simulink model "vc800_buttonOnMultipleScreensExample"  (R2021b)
settings: Solver=FixedStepDiscrete  StartTime=0.0  StopTime=10.0  FixedStep=0.01  RelTol=1e-3  EnableMultiTasking=on
PreLoadFcn:
  | try, model_open; catch, disp('Error occurred while executing model pre-load callback: model_open.m'); disp('Please assure that the MATLAB working directory is set to the model directory before opening.'); end
InitFcn:
  | try, model_open; catch, end
model workspace (MAT data in the model file):
  IOScreen_Label_XCoord = 1
  IOScreen_Row1_YCoord = 1
  IOScreen_Row2_YCoord = 12
  IOScreen_Value_XCoord = 110
  MainScreen_Row1_YCoord = 7
  MainScreen_Row2_YCoord = 23
  MainScreen_Symbols_XCoord = 1
  MainScreen_Units_XCoord = 69
  MainScreen_Value_XCoord = 64
undefined symbols (not defined in the file or in its folder): case, curr_screen, default, DISP, filtering, gesture, hex2dec, Mode, No, raptor_get_buildNum, raptor_get_safe_string, raptor_hwexp, raptor_xcp_function, Screens, VC800, Voltage
libraries: Raptor_display_lib x190, Raptor_lib x97, simulink_extras x11, Raptor_Datalogging_lib x10, simulink x2
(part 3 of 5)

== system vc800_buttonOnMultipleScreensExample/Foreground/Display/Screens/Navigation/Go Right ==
  Current Screen : Inport
  Action Port : ActionPort  ActionPortLabel=if(u1 == 3)
  About : Subsystem  TreatAsAtomicUnit=on
  DataLog : Subsystem  TreatAsAtomicUnit=on
  Default : Subsystem  TreatAsAtomicUnit=on
  Input : Subsystem  TreatAsAtomicUnit=on
  Main : Subsystem  TreatAsAtomicUnit=on
  Ouptut : Subsystem  TreatAsAtomicUnit=on
  Switch Case : SwitchCase  CaseConditions={1,2,3,4,5}
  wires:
  Current Screen/1 -> Switch Case/1
  Switch Case/1 -> Main/Action
  Switch Case/4 -> DataLog/Action
  Switch Case/5 -> About/Action
  Switch Case/2 -> Input/Action
  Switch Case/6 -> Default/Action
  Switch Case/3 -> Ouptut/Action

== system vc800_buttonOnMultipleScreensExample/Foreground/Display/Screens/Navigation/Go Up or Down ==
  note: Do Nothing when a "UP" or "DOWN" is performed
  Current Screen : Inport
  Action Port : ActionPort  ActionPortLabel=else
  Terminator : Terminator
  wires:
  Current Screen/1 -> Terminator/1

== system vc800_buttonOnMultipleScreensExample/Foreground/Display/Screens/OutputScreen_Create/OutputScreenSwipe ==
  note: This function is called when a swipe action occurs. The gesture input will provide the gesture detected: 0 = UP 1 = DOWN 2 = LEFT 3 = RIGHT
  OutputScreenSwipe : TriggerPort  TriggerType=function-call  IsSimulinkFunction=on  FunctionName=OutputScreenSwipe  FunctionVisibility=scoped  VariantControl=Variant  PortDimensions=1
  Constant : Constant  Value=3  OutDataTypeStr=uint8
  Function Caller : FunctionCaller  FunctionPrototype=Screens.Navigation(gesture,curr_screen)  InputArgumentSpecifications=<Enter example>  OutputArgumentSpecifications=<Enter example>
  gesture : ArgIn  OutDataTypeStr=uint8  ArgumentName=gesture
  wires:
  gesture/1 -> Function Caller/1
  Constant/1 -> Function Caller/2

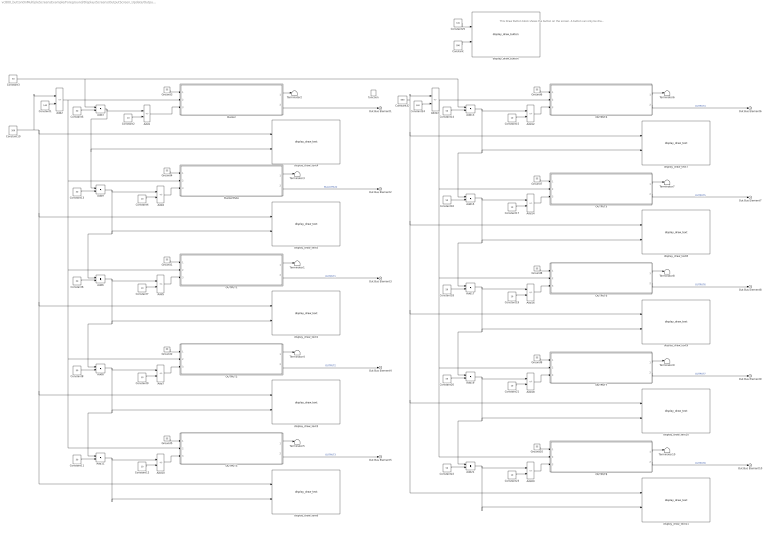
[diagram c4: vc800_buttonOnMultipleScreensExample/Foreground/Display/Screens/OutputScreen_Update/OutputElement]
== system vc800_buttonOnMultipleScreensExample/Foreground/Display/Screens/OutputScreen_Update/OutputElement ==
  note: This Draw Button block shows the button on the screen. A button can only be drawn once per screen.
  function : TriggerPort  TriggerType=function-call  VariantControl=Variant
  Add{1..2,4..5,7,10,12,14,16,18,20,22} (12 alike) : Sum  Inputs=+-
  Add{3,6,8..9,11,13,15,17,19,21} (10 alike) : Sum
  Buzzer : Subsystem  mask(Display Toggle){InitialCondition=0}
      mask prompts: InitialCondition "Initial Condition"
      mask help: Draws a toggle switch onto the screen that will hold either an off or an on state
  BuzzerMute : Subsystem  mask(Display Toggle){InitialCondition=0}
      mask prompts: InitialCondition "Initial Condition"
      mask help: Draws a toggle switch onto the screen that will hold either an off or an on state
  Constant : Constant  Value=390  OutDataTypeStr=Inherit: Inherit via back propagation
  Constant1 : Constant  Value=140  OutDataTypeStr=int32
  Constant10 : Constant  Value=200  OutDataTypeStr=int32
  Constant{3,5..6,8,11,13..14,16,18,20,22} (11 alike) : Constant  Value=50  OutDataTypeStr=int32
  Constant{2,4,7,9,12,15,17,19,21,23} (10 alike) : Constant  Value=10  OutDataTypeStr=int32
  Constant24 : Constant  Value=140  OutDataTypeStr=int32
  Constant25 : Constant  Value=720  OutDataTypeStr=Inherit: Inherit via back propagation
  Constant32 : Constant  Value=600  OutDataTypeStr=int32
  Ground{1..10} (10 alike) : Ground
  OUTPUT1 : Subsystem  mask(Display Toggle){InitialCondition=0}
      mask prompts: InitialCondition "Initial Condition"
      mask help: Draws a toggle switch onto the screen that will hold either an off or an on state
  OUTPUT2 : Subsystem  mask(Display Toggle){InitialCondition=0}
      mask prompts: InitialCondition "Initial Condition"
      mask help: Draws a toggle switch onto the screen that will hold either an off or an on state
  OUTPUT3 : Subsystem  mask(Display Toggle){InitialCondition=0}
      mask prompts: InitialCondition "Initial Condition"
      mask help: Draws a toggle switch onto the screen that will hold either an off or an on state
  OUTPUT4 : Subsystem  mask(Display Toggle){InitialCondition=0}
      mask prompts: InitialCondition "Initial Condition"
      mask help: Draws a toggle switch onto the screen that will hold either an off or an on state
  OUTPUT5 : Subsystem  mask(Display Toggle){InitialCondition=0}
      mask prompts: InitialCondition "Initial Condition"
      mask help: Draws a toggle switch onto the screen that will hold either an off or an on state
  OUTPUT6 : Subsystem  mask(Display Toggle){InitialCondition=0}
      mask prompts: InitialCondition "Initial Condition"
      mask help: Draws a toggle switch onto the screen that will hold either an off or an on state
  OUTPUT7 : Subsystem  mask(Display Toggle){InitialCondition=0}
      mask prompts: InitialCondition "Initial Condition"
      mask help: Draws a toggle switch onto the screen that will hold either an off or an on state
  OUTPUT8 : Subsystem  mask(Display Toggle){InitialCondition=0}
      mask prompts: InitialCondition "Initial Condition"
      mask help: Draws a toggle switch onto the screen that will hold either an off or an on state
  Terminator{1..10} (10 alike) : Terminator
  display_draw_button : Raptor_display_lib/Drawing Functions/display_draw_button  ButtonName='GoToAbout'
  display_draw_text1 : Raptor_display_lib/Drawing Functions/display_draw_text  textPort=off  textVal='OUTPUT1'  colorPort=off  col=FFFF  opacity=100  font=Future  fontFile=''  heightPort=off  height=20  hAlign=Left  vAlign=Top  spacing=0  layer=Background  pnPort=off
  display_draw_text10 : Raptor_display_lib/Drawing Functions/display_draw_text  textPort=off  textVal='OUTPUT7'  colorPort=off  col=FFFF  opacity=100  font=Future  fontFile=''  heightPort=off  height=20  hAlign=Left  vAlign=Top  spacing=0  layer=Background  pnPort=off
  display_draw_text11 : Raptor_display_lib/Drawing Functions/display_draw_text  textPort=off  textVal='OUTPUT8'  colorPort=off  col=FFFF  opacity=100  font=Future  fontFile=''  heightPort=off  height=20  hAlign=Left  vAlign=Top  spacing=0  layer=Background  pnPort=off
  display_draw_text3 : Raptor_display_lib/Drawing Functions/display_draw_text  textPort=off  textVal='OUTPUT2'  colorPort=off  col=FFFF  opacity=100  font=Future  fontFile=''  heightPort=off  height=20  hAlign=Left  vAlign=Top  spacing=0  layer=Background  pnPort=off
  display_draw_text4 : Raptor_display_lib/Drawing Functions/display_draw_text  textPort=off  textVal='Buzzer'  colorPort=off  col=FFFF  opacity=100  font=Future  fontFile=''  heightPort=off  height=20  hAlign=Left  vAlign=Top  spacing=0  layer=Background  pnPort=off
  display_draw_text5 : Raptor_display_lib/Drawing Functions/display_draw_text  textPort=off  textVal='Buzzer Mute'  colorPort=off  col=FFFF  opacity=100  font=Future  fontFile=''  heightPort=off  height=20  hAlign=Left  vAlign=Top  spacing=0  layer=Background  pnPort=off
  display_draw_text6 : Raptor_display_lib/Drawing Functions/display_draw_text  textPort=off  textVal='OUTPUT3'  colorPort=off  col=FFFF  opacity=100  font=Future  fontFile=''  heightPort=off  height=20  hAlign=Left  vAlign=Top  spacing=0  layer=Background  pnPort=off
  display_draw_text7 : Raptor_display_lib/Drawing Functions/display_draw_text  textPort=off  textVal='OUTPUT4'  colorPort=off  col=FFFF  opacity=100  font=Future  fontFile=''  heightPort=off  height=20  hAlign=Left  vAlign=Top  spacing=0  layer=Background  pnPort=off
  display_draw_text8 : Raptor_display_lib/Drawing Functions/display_draw_text  textPort=off  textVal='OUTPUT5'  colorPort=off  col=FFFF  opacity=100  font=Future  fontFile=''  heightPort=off  height=20  hAlign=Left  vAlign=Top  spacing=0  layer=Background  pnPort=off
  display_draw_text9 : Raptor_display_lib/Drawing Functions/display_draw_text  textPort=off  textVal='OUTPUT6'  colorPort=off  col=FFFF  opacity=100  font=Future  fontFile=''  heightPort=off  height=20  hAlign=Left  vAlign=Top  spacing=0  layer=Background  pnPort=off
  Out Bus Element{1..10} (10 alike) : Outport  VectorParamsAs1DForOutWhenUnconnected=off
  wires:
  Add20/1 -> OUTPUT8/3(y)
  Constant23/1 -> Add20/2
  Add19/1 -> Add18/1, Add21/1, display_draw_text10/2
  Add2/1 -> BuzzerMute/2(x), OUTPUT1/2(x), OUTPUT2/2(x), OUTPUT3/2(x), Buzzer/2(x)
  Constant10/1 -> Add2/1, display_draw_text5/1, display_draw_text1/1, display_draw_text3/1, display_draw_text6/1, display_draw_text4/1
  OUTPUT8/2(out) -> Out Bus Element10/1  "OUTPUT8"
  OUTPUT8/1(next) -> Terminator10/1
  Add21/1 -> display_draw_text11/2, Add20/1
  Ground10/1 -> OUTPUT8/1(prev)
  Constant22/1 -> Add21/2
  Constant20/1 -> Add19/2
  Ground9/1 -> OUTPUT7/1(prev)
  OUTPUT7/1(next) -> Terminator9/1
  OUTPUT7/2(out) -> Out Bus Element9/1  "OUTPUT7"
  Add17/1 -> display_draw_text9/2, Add19/1, Add16/1
  Constant21/1 -> Add18/2
  Add18/1 -> OUTPUT7/3(y)
  Add16/1 -> OUTPUT6/3(y)
  Constant19/1 -> Add16/2
  Add15/1 -> Add14/1, Add17/1, display_draw_text8/2
  OUTPUT6/2(out) -> Out Bus Element8/1  "OUTPUT6"
  OUTPUT6/1(next) -> Terminator8/1
  Ground8/1 -> OUTPUT6/1(prev)
  Constant18/1 -> Add17/2
  Constant16/1 -> Add15/2
  Ground7/1 -> OUTPUT5/1(prev)
  OUTPUT5/1(next) -> Terminator7/1
  OUTPUT5/2(out) -> Out Bus Element7/1  "OUTPUT5"
  Add13/1 -> Add15/1, display_draw_text7/2, Add12/1
  Constant17/1 -> Add14/2
  Add14/1 -> OUTPUT5/3(y)
  Add12/1 -> OUTPUT4/3(y)
  Constant15/1 -> Add12/2
  Add11/1 -> display_draw_text6/2, Add10/1
  OUTPUT4/2(out) -> Out Bus Element6/1  "OUTPUT4"
  OUTPUT4/1(next) -> Terminator6/1
  Ground6/1 -> OUTPUT4/1(prev)
  Constant14/1 -> Add13/2
  Constant11/1 -> Add11/2
  Ground5/1 -> OUTPUT3/1(prev)
  OUTPUT3/1(next) -> Terminator5/1
  OUTPUT3/2(out) -> Out Bus Element5/1  "OUTPUT3"
  Add8/1 -> display_draw_text3/2, Add11/1, Add7/1
  Constant12/1 -> Add10/2
  Add10/1 -> OUTPUT3/3(y)
  Add7/1 -> OUTPUT2/3(y)
  Constant9/1 -> Add7/2
  Add6/1 -> Add5/1, display_draw_text1/2, Add8/1
  OUTPUT2/2(out) -> Out Bus Element4/1  "OUTPUT2"
  OUTPUT2/1(next) -> Terminator4/1
  Ground2/1 -> OUTPUT2/1(prev)
  Constant8/1 -> Add8/2
  Constant6/1 -> Add6/2
  Ground1/1 -> OUTPUT1/1(prev)
  OUTPUT1/1(next) -> Terminator1/1
  OUTPUT1/2(out) -> Out Bus Element3/1  "OUTPUT1"
  Add9/1 -> Add6/1, display_draw_text5/2, Add4/1
  Constant7/1 -> Add5/2
  Add5/1 -> OUTPUT1/3(y)
  Add4/1 -> BuzzerMute/3(y)
  Constant4/1 -> Add4/2
  Add1/1 -> Buzzer/3(y)
  Constant2/1 -> Add1/2
  Constant5/1 -> Add3/2
  Add3/1 -> Add9/1, display_draw_text4/2, Add1/1
  Constant1/1 -> Add2/2
  Constant3/1 -> Add3/1, Add13/1
  Ground3/1 -> Buzzer/1(prev)
  Buzzer/1(next) -> Terminator2/1
  Buzzer/2(out) -> Out Bus Element1/1
  BuzzerMute/2(out) -> Out Bus Element2/1  "BuzzerMute"
  BuzzerMute/1(next) -> Terminator3/1
  Ground4/1 -> BuzzerMute/1(prev)
  Constant13/1 -> Add9/2
  Constant32/1 -> Add22/1, display_draw_text7/1, display_draw_text8/1, display_draw_text9/1, display_draw_text10/1, display_draw_text11/1
  Constant24/1 -> Add22/2
  Add22/1 -> OUTPUT4/2(x), OUTPUT8/2(x), OUTPUT7/2(x), OUTPUT6/2(x), OUTPUT5/2(x)
  Constant25/1 -> display_draw_button/1
  Constant/1 -> display_draw_button/2

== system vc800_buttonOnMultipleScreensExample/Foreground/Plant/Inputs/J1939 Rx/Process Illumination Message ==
  note: default to 100% illumination
  note: timeout occurred
  note: new message
  AgeCount : Inport
  Data : Inport  Port=2
  Constant : Constant  Value=750
  Constant1 : Constant  Value=0
  Constant2 : Constant  Value=100
  Constant3 : Constant  Value=100
  Logical Operator : Logic  Operator=NOT  AllPortsSameDT=off  OutDataTypeStr=boolean
  Logical Operator1 : Logic  Operator=OR  AllPortsSameDT=off  OutDataTypeStr=boolean
  Relational Operator : RelationalOperator  Operator=>  OutDataTypeStr=boolean  RndMeth=Simplest
  Relational Operator1 : RelationalOperator  Operator===  OutDataTypeStr=boolean  RndMeth=Simplest
  Relational Operator2 : RelationalOperator  Operator=>  OutDataTypeStr=boolean  RndMeth=Simplest
  Switch : Switch  Criteria=u2 ~= 0
  Switch1 : Switch  Criteria=u2 ~= 0
  Unit Delay : UnitDelay  SampleTime=-1  HasFrameUpgradeWarning=on
  Illumination : Outport  VectorParamsAs1DForOutWhenUnconnected=off
  IlluminationValid : Outport  Port=2  VectorParamsAs1DForOutWhenUnconnected=off
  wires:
  Constant/1 -> Relational Operator/2
  Logical Operator/1 -> IlluminationValid/1
  Switch/1 -> Illumination/1, Unit Delay/1
  AgeCount/1 -> Relational Operator1/1, Relational Operator/1
  Constant1/1 -> Relational Operator1/2
  Relational Operator1/1 -> Switch1/2
  Data/1 -> Switch1/1, Relational Operator2/1
  Switch1/1 -> Switch/3
  Unit Delay/1 -> Switch1/3
  Constant2/1 -> Switch/1
  Relational Operator/1 -> Logical Operator1/1
  Logical Operator1/1 -> Switch/2, Logical Operator/1
  Relational Operator2/1 -> Logical Operator1/2
  Constant3/1 -> Relational Operator2/2

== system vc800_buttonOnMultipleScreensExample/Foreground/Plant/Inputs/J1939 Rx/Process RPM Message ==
  note: timeout occurred
  note: new message
  AgeCount : Inport
  Data : Inport  Port=2
  Constant : Constant  Value=100
  Constant1 : Constant  Value=0
  Constant2 : Constant  Value=0
  Constant3 : Constant  Value=8031.88
  Logical Operator : Logic  Operator=NOT  AllPortsSameDT=off  OutDataTypeStr=boolean
  Logical Operator1 : Logic  Operator=OR  AllPortsSameDT=off  OutDataTypeStr=boolean
  Relational Operator : RelationalOperator  Operator=>  OutDataTypeStr=boolean  RndMeth=Simplest
  Relational Operator1 : RelationalOperator  Operator===  OutDataTypeStr=boolean  RndMeth=Simplest
  Relational Operator2 : RelationalOperator  Operator=>  OutDataTypeStr=boolean  RndMeth=Simplest
  Switch : Switch  Criteria=u2 ~= 0
  Switch1 : Switch  Criteria=u2 ~= 0
  Unit Delay : UnitDelay  SampleTime=-1  HasFrameUpgradeWarning=on
  EngineRPM : Outport  VectorParamsAs1DForOutWhenUnconnected=off
  EngineRPMValid : Outport  Port=2  VectorParamsAs1DForOutWhenUnconnected=off
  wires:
  Constant/1 -> Relational Operator/2
  Logical Operator/1 -> EngineRPMValid/1
  Switch/1 -> EngineRPM/1, Unit Delay/1
  AgeCount/1 -> Relational Operator1/1, Relational Operator/1
  Constant1/1 -> Relational Operator1/2
  Relational Operator1/1 -> Switch1/2
  Data/1 -> Switch1/1, Relational Operator2/1
  Switch1/1 -> Switch/3
  Unit Delay/1 -> Switch1/3
  Constant2/1 -> Switch/1
  Relational Operator/1 -> Logical Operator1/1
  Logical Operator1/1 -> Switch/2, Logical Operator/1
  Relational Operator2/1 -> Logical Operator1/2
  Constant3/1 -> Relational Operator2/2

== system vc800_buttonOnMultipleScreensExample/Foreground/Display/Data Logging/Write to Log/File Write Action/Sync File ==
  In1 : Inport
  Enable : EnablePort
  Terminator : Terminator
  Terminator1 : Terminator
  raptor_data_write : Raptor_lib/Data Storage/raptor_data_write  dataName='LastSync'  dataShape=Scalar  idxSource=Input Port  idxRow=1  idxCol=1
  raptor_fileIO_sync1 : Raptor_Datalogging_lib/raptor_fileIO_sync  resourceValues=USB|(None)  resource=USB
  raptor_time : Raptor_lib/Triggers/raptor_time  unit=milliseconds
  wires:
  raptor_time/1 -> raptor_data_write/1
  raptor_fileIO_sync1/1 -> Terminator/1
  In1/1 -> raptor_fileIO_sync1/1
  raptor_fileIO_sync1/2 -> Terminator1/1

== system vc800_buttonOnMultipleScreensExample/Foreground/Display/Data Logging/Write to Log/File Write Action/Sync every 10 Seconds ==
  Add1 : Sum  Inputs=+-
  Constant : Constant  Value=10000
  Logical Operator : Logic  Operator=OR  AllPortsSameDT=off  OutDataTypeStr=boolean
  Relational Operator : RelationalOperator  Operator=>  OutDataTypeStr=boolean
  Relational Operator1 : RelationalOperator  Operator=<  OutDataTypeStr=boolean
  Unit Delay : UnitDelay  SampleTime=-1  HasFrameUpgradeWarning=on
  raptor_data_def : Raptor_lib/Data Storage/raptor_data_def  dataName='LastSync'  initValue=0  dataType=uint32  storage=Volatile (RAM)  calVisible=on  calType=Measurement  calDispType=Number  calEnum={'False', 'True'}  calGain=1.0  calOffset=0  calMin=-Inf  calMax=Inf  calFormat='4.2'  calUnit=''  calHelp=['Block:' gcb]  calAccess=4  calFunction=raptor_xcp_function(gcb)  calDispHeaders=off  calColHeaders={'Col1' 'Col2' 'Col3'}  calRowHeaders={'Row1' 'Row2' 'Row3'}
  raptor_data_read1 : Raptor_lib/Data Storage/raptor_data_read  dataName='LastSync'  dataShape=Scalar  idxSource=Input  idxRow=1  idxCol=1
  raptor_time : Raptor_lib/Triggers/raptor_time  unit=milliseconds
  TimeToSync : Outport  VectorParamsAs1DForOutWhenUnconnected=off
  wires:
  Logical Operator/1 -> TimeToSync/1
  Relational Operator1/1 -> Logical Operator/2  "Rollover"
  Relational Operator/1 -> Logical Operator/1
  Constant/1 -> Relational Operator/2
  Add1/1 -> Relational Operator/1
  raptor_data_read1/1 -> Add1/2
  Unit Delay/1 -> Relational Operator1/2
  raptor_time/1 -> Relational Operator1/1, Add1/1, Unit Delay/1

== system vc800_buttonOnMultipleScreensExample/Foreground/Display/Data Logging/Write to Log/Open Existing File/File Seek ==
  Open File Handle : Inport
  Open Success : Inport  Port=2
  File Open Failure : Subsystem
  File Open Success : Subsystem
  Logical Operator : Logic  Operator=NOT  AllPortsSameDT=off  OutDataTypeStr=boolean
  Seek File Handle Success : Outport  VectorParamsAs1DForOutWhenUnconnected=off
  Seek Success : Outport  Port=2  VectorParamsAs1DForOutWhenUnconnected=off
  Seek File Handle Failure : Outport  Port=3  VectorParamsAs1DForOutWhenUnconnected=off
  Seek Failure : Outport  Port=4  VectorParamsAs1DForOutWhenUnconnected=off
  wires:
  Open File Handle/1 -> File Open Success/1(file_in), File Open Failure/1(file_in)
  Logical Operator/1 -> File Open Failure/Enable
  Open Success/1 -> Logical Operator/1, File Open Success/Enable
  File Open Success/1(file_out) -> Seek File Handle Success/1
  File Open Success/2(Out2) -> Seek Success/1
  File Open Failure/1(file_out) -> Seek File Handle Failure/1
  File Open Failure/2(Success) -> Seek Failure/1

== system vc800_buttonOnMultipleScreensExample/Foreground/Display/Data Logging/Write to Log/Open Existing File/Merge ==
  File Handle Success : Inport
  File Open Success : Inport  Port=2
  File Handle Failure : Inport  Port=3
  File Open Failure : Inport  Port=4
  Merge : Merge
  Merge1 : Merge
  Handle : Outport  VectorParamsAs1DForOutWhenUnconnected=off
  Success : Outport  Port=2  VectorParamsAs1DForOutWhenUnconnected=off
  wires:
  Merge1/1 -> Handle/1
  Merge/1 -> Success/1
  File Open Failure/1 -> Merge/2
  File Handle Failure/1 -> Merge1/2
  File Handle Success/1 -> Merge1/1
  File Open Success/1 -> Merge/1

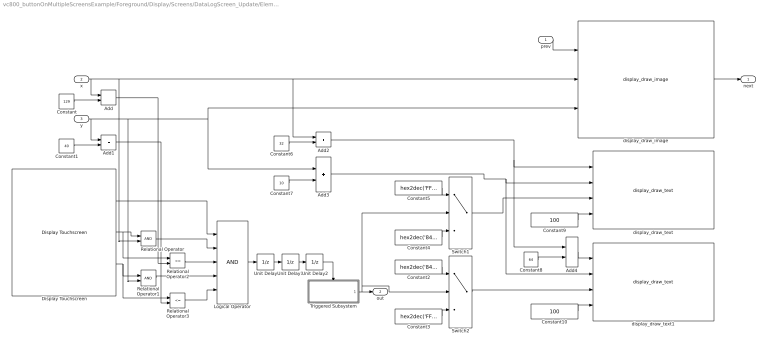
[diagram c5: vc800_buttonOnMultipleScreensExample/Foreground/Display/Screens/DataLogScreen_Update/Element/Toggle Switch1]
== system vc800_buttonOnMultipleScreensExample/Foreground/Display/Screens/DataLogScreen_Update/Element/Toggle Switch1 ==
  prev : Inport
  x : Inport  Port=2
  y : Inport  Port=3
  Add{,1..4} (5 alike) : Sum
  Constant : Constant  Value=129
  Constant1 : Constant  Value=40
  Constant10 : Constant  Value=100  OutDataTypeStr=uint32
  Constant2 : Constant  Value=hex2dec('8410')  OutDataTypeStr=uint16
  Constant3 : Constant  Value=hex2dec('FFFF')  OutDataTypeStr=uint16
  Constant4 : Constant  Value=hex2dec('8410')  OutDataTypeStr=uint16
  Constant5 : Constant  Value=hex2dec('FFFF')  OutDataTypeStr=uint16
  Constant6 : Constant  Value=32  OutDataTypeStr=int32
  Constant7 : Constant  Value=10  OutDataTypeStr=int32
  Constant8 : Constant  Value=64  OutDataTypeStr=int32
  Constant9 : Constant  Value=100  OutDataTypeStr=uint32
  Display Touchscreen : Raptor_display_lib/Touchscreen/Display Touchscreen
  Logical Operator : Logic  Inputs=5  IconShape=distinctive  AllPortsSameDT=off  OutDataTypeStr=boolean
  Relational Operator : RelationalOperator  OutDataTypeStr=boolean
  Relational Operator1 : RelationalOperator  OutDataTypeStr=boolean
  Relational Operator2 : RelationalOperator  Operator=<=  OutDataTypeStr=boolean
  Relational Operator3 : RelationalOperator  Operator=<=  OutDataTypeStr=boolean
  Switch1 : Switch  Criteria=u2 ~= 0
  Switch2 : Switch  Criteria=u2 ~= 0
  Triggered Subsystem : Subsystem  TreatAsAtomicUnit=on
  Unit Delay : UnitDelay  SampleTime=-1  HasFrameUpgradeWarning=on
  Unit Delay1 : UnitDelay  InitialCondition=1  SampleTime=-1  HasFrameUpgradeWarning=on
  Unit Delay2 : UnitDelay  SampleTime=-1  HasFrameUpgradeWarning=on
  display_draw_image : Raptor_display_lib/Drawing Functions/display_draw_image  imagePort=off  imageFile=toggle_frame.png  opacityPort=off  opacity=100  drawMode=Draw Entire Image  alpha=Draw as Transparent  layer=Background  drawModeXY=Top Left  pnPort=on
  display_draw_text : Raptor_display_lib/Drawing Functions/display_draw_text  textPort=off  textVal='On'  colorPort=on  col=8410  opacity=100  font=Future  fontFile=''  heightPort=off  height=20  hAlign=Center  vAlign=Top  spacing=0  layer=Background  pnPort=off
  display_draw_text1 : Raptor_display_lib/Drawing Functions/display_draw_text  textPort=off  textVal='Off'  colorPort=on  col=FFFF  opacity=100  font=Future  fontFile=''  heightPort=off  height=20  hAlign=Center  vAlign=Top  spacing=0  layer=Background  pnPort=off
  next : Outport  VectorParamsAs1DForOutWhenUnconnected=off
  out : Outport  Port=2  VectorParamsAs1DForOutWhenUnconnected=off
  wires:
  x/1 -> Add/1, Relational Operator/2, Add2/1, display_draw_image/2
  Display Touchscreen/2 -> Relational Operator/1, Relational Operator2/1
  Display Touchscreen/3 -> Relational Operator1/1, Relational Operator3/1
  y/1 -> Add1/1, Relational Operator1/2, Add3/1, display_draw_image/3
  Constant/1 -> Add/2
  Constant1/1 -> Add1/2
  Add/1 -> Relational Operator2/2
  Add1/1 -> Relational Operator3/2
  Relational Operator3/1 -> Logical Operator/5
  Relational Operator1/1 -> Logical Operator/4
  Relational Operator2/1 -> Logical Operator/3
  Relational Operator/1 -> Logical Operator/2
  Display Touchscreen/1 -> Logical Operator/1
  Unit Delay1/1 -> Unit Delay2/1
  Unit Delay/1 -> Unit Delay1/1
  Logical Operator/1 -> Unit Delay/1
  Unit Delay2/1 -> Triggered Subsystem/Trigger
  prev/1 -> display_draw_image/1
  display_draw_image/1 -> next/1
  Triggered Subsystem/1(Out1) -> Switch1/2, Switch2/2, out/1
  Switch1/1 -> display_draw_text/3
  Switch2/1 -> display_draw_text1/3
  Constant2/1 -> Switch2/1
  Constant4/1 -> Switch1/3
  Constant3/1 -> Switch2/3
  Constant5/1 -> Switch1/1
  Constant6/1 -> Add2/2
  Add2/1 -> Add4/1, display_draw_text/1
  Constant7/1 -> Add3/2
  Add3/1 -> display_draw_text/2, display_draw_text1/2
  Constant8/1 -> Add4/2
  Add4/1 -> display_draw_text1/1
  Constant9/1 -> display_draw_text/4
  Constant10/1 -> display_draw_text1/4

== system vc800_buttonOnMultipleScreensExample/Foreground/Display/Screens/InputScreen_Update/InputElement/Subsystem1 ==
  y_start_offset : Inport
  x : Inport  Port=2
  In3 : Inport  Port=3
  in_value : Inport  Port=4
  Add22 : Sum
  Constant26 : Constant  Value=40  OutDataTypeStr=int32
  display_draw_text13 : Raptor_display_lib/Drawing Functions/display_draw_text  textPort=off  textVal=in_nam  colorPort=off  col=FFFF  opacity=100  font=Future  fontFile=''  heightPort=off  height=20  hAlign=Right  vAlign=Center  spacing=0  layer=Background  pnPort=off
  display_draw_text14 : Raptor_display_lib/Drawing Functions/display_draw_text  textPort=on  textVal='Input1'  colorPort=off  col=FFFF  opacity=100  font=Future  fontFile=''  heightPort=off  height=20  hAlign=Left  vAlign=Center  spacing=0  layer=Background  pnPort=off
  raptor_string : Raptor_lib/Strings/raptor_string  stringName=''  string=''  dynamicSize=Fixed Size  strSize=10  storage=Volatile (RAM)  calVisible=off  calAccess=4  strFunction=raptor_xcp_function(gcb)
  raptor_string_printf : Raptor_lib/Strings/raptor_string_printf  formatString='%u'
  y_end_offset : Outport  VectorParamsAs1DForOutWhenUnconnected=off
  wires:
  raptor_string/1 -> raptor_string_printf/1
  Add22/1 -> display_draw_text13/2, y_end_offset/1, display_draw_text14/2
  In3/1 -> display_draw_text14/1
  raptor_string_printf/1 -> display_draw_text14/3
  y_start_offset/1 -> Add22/1
  Constant26/1 -> Add22/2
  in_value/1 -> raptor_string_printf/2
  x/1 -> display_draw_text13/1

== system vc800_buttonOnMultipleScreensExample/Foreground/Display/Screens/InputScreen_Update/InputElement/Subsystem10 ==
  y_start_offset : Inport
  x : Inport  Port=2
  In3 : Inport  Port=3
  in_value : Inport  Port=4
  Add22 : Sum
  Constant26 : Constant  Value=40  OutDataTypeStr=int32
  display_draw_text13 : Raptor_display_lib/Drawing Functions/display_draw_text  textPort=off  textVal=in_nam  colorPort=off  col=FFFF  opacity=100  font=Future  fontFile=''  heightPort=off  height=20  hAlign=Right  vAlign=Center  spacing=0  layer=Background  pnPort=off
  display_draw_text14 : Raptor_display_lib/Drawing Functions/display_draw_text  textPort=on  textVal='Input1'  colorPort=off  col=FFFF  opacity=100  font=Future  fontFile=''  heightPort=off  height=20  hAlign=Left  vAlign=Center  spacing=0  layer=Background  pnPort=off
  raptor_string : Raptor_lib/Strings/raptor_string  stringName=''  string=''  dynamicSize=Fixed Size  strSize=10  storage=Volatile (RAM)  calVisible=off  calAccess=4  strFunction=raptor_xcp_function(gcb)
  raptor_string_printf : Raptor_lib/Strings/raptor_string_printf  formatString='%u'
  y_end_offset : Outport  VectorParamsAs1DForOutWhenUnconnected=off
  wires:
  x/1 -> display_draw_text13/1
  in_value/1 -> raptor_string_printf/2
  Constant26/1 -> Add22/2
  y_start_offset/1 -> Add22/1
  raptor_string_printf/1 -> display_draw_text14/3
  In3/1 -> display_draw_text14/1
  Add22/1 -> display_draw_text14/2, y_end_offset/1, display_draw_text13/2
  raptor_string/1 -> raptor_string_printf/1

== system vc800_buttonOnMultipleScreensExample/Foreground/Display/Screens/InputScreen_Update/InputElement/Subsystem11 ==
  y_start_offset : Inport
  x : Inport  Port=2
  In3 : Inport  Port=3
  in_value : Inport  Port=4
  Add22 : Sum
  Constant26 : Constant  Value=40  OutDataTypeStr=int32
  display_draw_text13 : Raptor_display_lib/Drawing Functions/display_draw_text  textPort=off  textVal=in_nam  colorPort=off  col=FFFF  opacity=100  font=Future  fontFile=''  heightPort=off  height=20  hAlign=Right  vAlign=Center  spacing=0  layer=Background  pnPort=off
  display_draw_text14 : Raptor_display_lib/Drawing Functions/display_draw_text  textPort=on  textVal='Input1'  colorPort=off  col=FFFF  opacity=100  font=Future  fontFile=''  heightPort=off  height=20  hAlign=Left  vAlign=Center  spacing=0  layer=Background  pnPort=off
  raptor_string : Raptor_lib/Strings/raptor_string  stringName=''  string=''  dynamicSize=Fixed Size  strSize=10  storage=Volatile (RAM)  calVisible=off  calAccess=4  strFunction=raptor_xcp_function(gcb)
  raptor_string_printf : Raptor_lib/Strings/raptor_string_printf  formatString='%u'
  y_end_offset : Outport  VectorParamsAs1DForOutWhenUnconnected=off
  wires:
  raptor_string/1 -> raptor_string_printf/1
  Add22/1 -> display_draw_text13/2, y_end_offset/1, display_draw_text14/2
  In3/1 -> display_draw_text14/1
  raptor_string_printf/1 -> display_draw_text14/3
  y_start_offset/1 -> Add22/1
  Constant26/1 -> Add22/2
  in_value/1 -> raptor_string_printf/2
  x/1 -> display_draw_text13/1

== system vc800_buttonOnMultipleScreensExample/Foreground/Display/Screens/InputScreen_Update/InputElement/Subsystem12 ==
  y_start_offset : Inport
  x : Inport  Port=2
  In3 : Inport  Port=3
  in_value : Inport  Port=4
  Add22 : Sum
  Constant26 : Constant  Value=40  OutDataTypeStr=int32
  display_draw_text13 : Raptor_display_lib/Drawing Functions/display_draw_text  textPort=off  textVal=in_nam  colorPort=off  col=FFFF  opacity=100  font=Future  fontFile=''  heightPort=off  height=20  hAlign=Right  vAlign=Center  spacing=0  layer=Background  pnPort=off
  display_draw_text14 : Raptor_display_lib/Drawing Functions/display_draw_text  textPort=on  textVal='Input1'  colorPort=off  col=FFFF  opacity=100  font=Future  fontFile=''  heightPort=off  height=20  hAlign=Left  vAlign=Center  spacing=0  layer=Background  pnPort=off
  raptor_string : Raptor_lib/Strings/raptor_string  stringName=''  string=''  dynamicSize=Fixed Size  strSize=10  storage=Volatile (RAM)  calVisible=off  calAccess=4  strFunction=raptor_xcp_function(gcb)
  raptor_string_printf : Raptor_lib/Strings/raptor_string_printf  formatString='%u'
  y_end_offset : Outport  VectorParamsAs1DForOutWhenUnconnected=off
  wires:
  x/1 -> display_draw_text13/1
  in_value/1 -> raptor_string_printf/2
  Constant26/1 -> Add22/2
  y_start_offset/1 -> Add22/1
  raptor_string_printf/1 -> display_draw_text14/3
  In3/1 -> display_draw_text14/1
  Add22/1 -> display_draw_text14/2, y_end_offset/1, display_draw_text13/2
  raptor_string/1 -> raptor_string_printf/1

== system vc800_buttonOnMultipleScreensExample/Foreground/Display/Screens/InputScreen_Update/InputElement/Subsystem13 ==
  y_start_offset : Inport
  x : Inport  Port=2
  In3 : Inport  Port=3
  in_value : Inport  Port=4
  Add22 : Sum
  Constant26 : Constant  Value=40  OutDataTypeStr=int32
  display_draw_text13 : Raptor_display_lib/Drawing Functions/display_draw_text  textPort=off  textVal=in_nam  colorPort=off  col=FFFF  opacity=100  font=Future  fontFile=''  heightPort=off  height=20  hAlign=Right  vAlign=Center  spacing=0  layer=Background  pnPort=off
  display_draw_text14 : Raptor_display_lib/Drawing Functions/display_draw_text  textPort=on  textVal='Input1'  colorPort=off  col=FFFF  opacity=100  font=Future  fontFile=''  heightPort=off  height=20  hAlign=Left  vAlign=Center  spacing=0  layer=Background  pnPort=off
  raptor_string : Raptor_lib/Strings/raptor_string  stringName=''  string=''  dynamicSize=Fixed Size  strSize=10  storage=Volatile (RAM)  calVisible=off  calAccess=4  strFunction=raptor_xcp_function(gcb)
  raptor_string_printf : Raptor_lib/Strings/raptor_string_printf  formatString='%u'
  y_end_offset : Outport  VectorParamsAs1DForOutWhenUnconnected=off
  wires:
  raptor_string/1 -> raptor_string_printf/1
  Add22/1 -> display_draw_text13/2, y_end_offset/1, display_draw_text14/2
  In3/1 -> display_draw_text14/1
  raptor_string_printf/1 -> display_draw_text14/3
  y_start_offset/1 -> Add22/1
  Constant26/1 -> Add22/2
  in_value/1 -> raptor_string_printf/2
  x/1 -> display_draw_text13/1

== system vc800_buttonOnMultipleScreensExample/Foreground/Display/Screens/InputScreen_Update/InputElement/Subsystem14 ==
  y_start_offset : Inport
  x : Inport  Port=2
  In3 : Inport  Port=3
  in_value : Inport  Port=4
  Add22 : Sum
  Constant26 : Constant  Value=40  OutDataTypeStr=int32
  display_draw_text13 : Raptor_display_lib/Drawing Functions/display_draw_text  textPort=off  textVal=in_nam  colorPort=off  col=FFFF  opacity=100  font=Future  fontFile=''  heightPort=off  height=20  hAlign=Right  vAlign=Center  spacing=0  layer=Background  pnPort=off
  display_draw_text14 : Raptor_display_lib/Drawing Functions/display_draw_text  textPort=on  textVal='Input1'  colorPort=off  col=FFFF  opacity=100  font=Future  fontFile=''  heightPort=off  height=20  hAlign=Left  vAlign=Center  spacing=0  layer=Background  pnPort=off
  raptor_string : Raptor_lib/Strings/raptor_string  stringName=''  string=''  dynamicSize=Fixed Size  strSize=10  storage=Volatile (RAM)  calVisible=off  calAccess=4  strFunction=raptor_xcp_function(gcb)
  raptor_string_printf : Raptor_lib/Strings/raptor_string_printf  formatString='%u'
  y_end_offset : Outport  VectorParamsAs1DForOutWhenUnconnected=off
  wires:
  x/1 -> display_draw_text13/1
  in_value/1 -> raptor_string_printf/2
  Constant26/1 -> Add22/2
  y_start_offset/1 -> Add22/1
  raptor_string_printf/1 -> display_draw_text14/3
  In3/1 -> display_draw_text14/1
  Add22/1 -> display_draw_text14/2, y_end_offset/1, display_draw_text13/2
  raptor_string/1 -> raptor_string_printf/1

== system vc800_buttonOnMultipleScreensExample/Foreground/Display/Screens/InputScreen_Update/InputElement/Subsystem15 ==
  y_start_offset : Inport
  x : Inport  Port=2
  x1 : Inport  Port=3
  in_value : Inport  Port=4
  Add1 : Sum
  Add22 : Sum
  Constant1 : Constant  Value=14  OutDataTypeStr=int32
  Constant26 : Constant  Value=40  OutDataTypeStr=int32
  Switch : Switch  Criteria=u2 ~= 0
  display_draw_image : Raptor_display_lib/Drawing Functions/display_draw_image  imagePort=on  imageFile=home.bmp  opacityPort=off  opacity=100  drawMode=Draw Entire Image  alpha=Draw as Transparent  layer=Background  drawModeXY=Center On Point  pnPort=off
  display_draw_text13 : Raptor_display_lib/Drawing Functions/display_draw_text  textPort=off  textVal=in_nam  colorPort=off  col=FFFF  opacity=100  font=Future  fontFile=''  heightPort=off  height=20  hAlign=Right  vAlign=Center  spacing=0  layer=Background  pnPort=off
  display_image_reference : Raptor_display_lib/Drawing Functions/display_image_reference  imageFile=Oval Driver.png
  display_image_reference1 : Raptor_display_lib/Drawing Functions/display_image_reference  imageFile=Oval Active.png
  y_end_offset : Outport  VectorParamsAs1DForOutWhenUnconnected=off
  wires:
  x/1 -> display_draw_text13/1
  in_value/1 -> Switch/2
  Constant26/1 -> Add22/2
  y_start_offset/1 -> Add22/1
  Add22/1 -> display_draw_image/2, y_end_offset/1, display_draw_text13/2
  display_image_reference/1 -> Switch/1
  display_image_reference1/1 -> Switch/3
  Switch/1 -> display_draw_image/3
  Constant1/1 -> Add1/2
  x1/1 -> Add1/1
  Add1/1 -> display_draw_image/1

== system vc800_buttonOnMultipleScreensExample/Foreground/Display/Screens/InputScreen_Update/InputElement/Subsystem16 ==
  y_start_offset : Inport
  x : Inport  Port=2
  x1 : Inport  Port=3
  in_value : Inport  Port=4
  Add1 : Sum
  Add22 : Sum
  Constant1 : Constant  Value=14  OutDataTypeStr=int32
  Constant26 : Constant  Value=40  OutDataTypeStr=int32
  Switch : Switch  Criteria=u2 ~= 0
  display_draw_image : Raptor_display_lib/Drawing Functions/display_draw_image  imagePort=on  imageFile=home.bmp  opacityPort=off  opacity=100  drawMode=Draw Entire Image  alpha=Draw as Transparent  layer=Background  drawModeXY=Center On Point  pnPort=off
  display_draw_text13 : Raptor_display_lib/Drawing Functions/display_draw_text  textPort=off  textVal=in_nam  colorPort=off  col=FFFF  opacity=100  font=Future  fontFile=''  heightPort=off  height=20  hAlign=Right  vAlign=Center  spacing=0  layer=Background  pnPort=off
  display_image_reference : Raptor_display_lib/Drawing Functions/display_image_reference  imageFile=Oval Driver.png
  display_image_reference1 : Raptor_display_lib/Drawing Functions/display_image_reference  imageFile=Oval Active.png
  y_end_offset : Outport  VectorParamsAs1DForOutWhenUnconnected=off
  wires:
  Add1/1 -> display_draw_image/1
  x1/1 -> Add1/1
  Constant1/1 -> Add1/2
  Switch/1 -> display_draw_image/3
  display_image_reference1/1 -> Switch/3
  display_image_reference/1 -> Switch/1
  Add22/1 -> display_draw_text13/2, y_end_offset/1, display_draw_image/2
  y_start_offset/1 -> Add22/1
  Constant26/1 -> Add22/2
  in_value/1 -> Switch/2
  x/1 -> display_draw_text13/1

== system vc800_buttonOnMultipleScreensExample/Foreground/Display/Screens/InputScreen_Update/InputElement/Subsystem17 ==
  y_start_offset : Inport
  x : Inport  Port=2
  x1 : Inport  Port=3
  in_value : Inport  Port=4
  Add1 : Sum
  Add22 : Sum
  Constant1 : Constant  Value=14  OutDataTypeStr=int32
  Constant26 : Constant  Value=40  OutDataTypeStr=int32
  Switch : Switch  Criteria=u2 ~= 0
  display_draw_image : Raptor_display_lib/Drawing Functions/display_draw_image  imagePort=on  imageFile=home.bmp  opacityPort=off  opacity=100  drawMode=Draw Entire Image  alpha=Draw as Transparent  layer=Background  drawModeXY=Center On Point  pnPort=off
  display_draw_text13 : Raptor_display_lib/Drawing Functions/display_draw_text  textPort=off  textVal=in_nam  colorPort=off  col=FFFF  opacity=100  font=Future  fontFile=''  heightPort=off  height=20  hAlign=Right  vAlign=Center  spacing=0  layer=Background  pnPort=off
  display_image_reference : Raptor_display_lib/Drawing Functions/display_image_reference  imageFile=Oval Driver.png
  display_image_reference1 : Raptor_display_lib/Drawing Functions/display_image_reference  imageFile=Oval Active.png
  y_end_offset : Outport  VectorParamsAs1DForOutWhenUnconnected=off
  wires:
  Add1/1 -> display_draw_image/1
  x1/1 -> Add1/1
  Constant1/1 -> Add1/2
  Switch/1 -> display_draw_image/3
  display_image_reference1/1 -> Switch/3
  display_image_reference/1 -> Switch/1
  Add22/1 -> display_draw_text13/2, y_end_offset/1, display_draw_image/2
  y_start_offset/1 -> Add22/1
  Constant26/1 -> Add22/2
  in_value/1 -> Switch/2
  x/1 -> display_draw_text13/1

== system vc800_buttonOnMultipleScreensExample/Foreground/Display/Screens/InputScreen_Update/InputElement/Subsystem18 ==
  y_start_offset : Inport
  x : Inport  Port=2
  In3 : Inport  Port=3
  in_value : Inport  Port=4
  Add22 : Sum
  Constant26 : Constant  Value=40  OutDataTypeStr=int32
  Data Type Conversion : DataTypeConversion  OutDataTypeStr=double
  display_draw_text13 : Raptor_display_lib/Drawing Functions/display_draw_text  textPort=off  textVal=in_nam  colorPort=off  col=FFFF  opacity=100  font=Future  fontFile=''  heightPort=off  height=20  hAlign=Right  vAlign=Center  spacing=0  layer=Background  pnPort=off
  display_draw_text14 : Raptor_display_lib/Drawing Functions/display_draw_text  textPort=on  textVal='Input1'  colorPort=off  col=FFFF  opacity=100  font=Future  fontFile=''  heightPort=off  height=20  hAlign=Left  vAlign=Center  spacing=0  layer=Background  pnPort=off
  raptor_string : Raptor_lib/Strings/raptor_string  stringName=''  string=''  dynamicSize=Fixed Size  strSize=10  storage=Volatile (RAM)  calVisible=off  calAccess=4  strFunction=raptor_xcp_function(gcb)
  raptor_string_printf : Raptor_lib/Strings/raptor_string_printf  formatString='%0.2f Hz'
  y_end_offset : Outport  VectorParamsAs1DForOutWhenUnconnected=off
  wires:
  raptor_string/1 -> raptor_string_printf/1
  Add22/1 -> display_draw_text13/2, y_end_offset/1, display_draw_text14/2
  In3/1 -> display_draw_text14/1
  raptor_string_printf/1 -> display_draw_text14/3
  y_start_offset/1 -> Add22/1
  Constant26/1 -> Add22/2
  in_value/1 -> Data Type Conversion/1
  x/1 -> display_draw_text13/1
  Data Type Conversion/1 -> raptor_string_printf/2

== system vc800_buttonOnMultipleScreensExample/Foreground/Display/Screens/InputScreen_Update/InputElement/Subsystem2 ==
  y_start_offset : Inport
  x : Inport  Port=2
  In3 : Inport  Port=3
  in_value : Inport  Port=4
  Add22 : Sum
  Constant26 : Constant  Value=40  OutDataTypeStr=int32
  display_draw_text13 : Raptor_display_lib/Drawing Functions/display_draw_text  textPort=off  textVal=in_nam  colorPort=off  col=FFFF  opacity=100  font=Future  fontFile=''  heightPort=off  height=20  hAlign=Right  vAlign=Center  spacing=0  layer=Background  pnPort=off
  display_draw_text14 : Raptor_display_lib/Drawing Functions/display_draw_text  textPort=on  textVal='Input1'  colorPort=off  col=FFFF  opacity=100  font=Future  fontFile=''  heightPort=off  height=20  hAlign=Left  vAlign=Center  spacing=0  layer=Background  pnPort=off
  raptor_string : Raptor_lib/Strings/raptor_string  stringName=''  string=''  dynamicSize=Fixed Size  strSize=10  storage=Volatile (RAM)  calVisible=off  calAccess=4  strFunction=raptor_xcp_function(gcb)
  raptor_string_printf : Raptor_lib/Strings/raptor_string_printf  formatString='%u'
  y_end_offset : Outport  VectorParamsAs1DForOutWhenUnconnected=off
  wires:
  raptor_string/1 -> raptor_string_printf/1
  Add22/1 -> display_draw_text13/2, y_end_offset/1, display_draw_text14/2
  In3/1 -> display_draw_text14/1
  raptor_string_printf/1 -> display_draw_text14/3
  y_start_offset/1 -> Add22/1
  Constant26/1 -> Add22/2
  in_value/1 -> raptor_string_printf/2
  x/1 -> display_draw_text13/1

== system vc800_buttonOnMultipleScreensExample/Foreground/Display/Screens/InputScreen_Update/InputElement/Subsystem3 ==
  y_start_offset : Inport
  x : Inport  Port=2
  In3 : Inport  Port=3
  in_value : Inport  Port=4
  Add22 : Sum
  Constant26 : Constant  Value=40  OutDataTypeStr=int32
  display_draw_text13 : Raptor_display_lib/Drawing Functions/display_draw_text  textPort=off  textVal=in_nam  colorPort=off  col=FFFF  opacity=100  font=Future  fontFile=''  heightPort=off  height=20  hAlign=Right  vAlign=Center  spacing=0  layer=Background  pnPort=off
  display_draw_text14 : Raptor_display_lib/Drawing Functions/display_draw_text  textPort=on  textVal='Input1'  colorPort=off  col=FFFF  opacity=100  font=Future  fontFile=''  heightPort=off  height=20  hAlign=Left  vAlign=Center  spacing=0  layer=Background  pnPort=off
  raptor_string : Raptor_lib/Strings/raptor_string  stringName=''  string=''  dynamicSize=Fixed Size  strSize=10  storage=Volatile (RAM)  calVisible=off  calAccess=4  strFunction=raptor_xcp_function(gcb)
  raptor_string_printf : Raptor_lib/Strings/raptor_string_printf  formatString='%u'
  y_end_offset : Outport  VectorParamsAs1DForOutWhenUnconnected=off
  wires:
  x/1 -> display_draw_text13/1
  in_value/1 -> raptor_string_printf/2
  Constant26/1 -> Add22/2
  y_start_offset/1 -> Add22/1
  raptor_string_printf/1 -> display_draw_text14/3
  In3/1 -> display_draw_text14/1
  Add22/1 -> display_draw_text14/2, y_end_offset/1, display_draw_text13/2
  raptor_string/1 -> raptor_string_printf/1

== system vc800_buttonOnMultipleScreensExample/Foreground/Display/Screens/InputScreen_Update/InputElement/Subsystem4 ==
  y_start_offset : Inport
  x : Inport  Port=2
  In3 : Inport  Port=3
  in_value : Inport  Port=4
  Add22 : Sum
  Constant26 : Constant  Value=40  OutDataTypeStr=int32
  display_draw_text13 : Raptor_display_lib/Drawing Functions/display_draw_text  textPort=off  textVal=in_nam  colorPort=off  col=FFFF  opacity=100  font=Future  fontFile=''  heightPort=off  height=20  hAlign=Right  vAlign=Center  spacing=0  layer=Background  pnPort=off
  display_draw_text14 : Raptor_display_lib/Drawing Functions/display_draw_text  textPort=on  textVal='Input1'  colorPort=off  col=FFFF  opacity=100  font=Future  fontFile=''  heightPort=off  height=20  hAlign=Left  vAlign=Center  spacing=0  layer=Background  pnPort=off
  raptor_string : Raptor_lib/Strings/raptor_string  stringName=''  string=''  dynamicSize=Fixed Size  strSize=10  storage=Volatile (RAM)  calVisible=off  calAccess=4  strFunction=raptor_xcp_function(gcb)
  raptor_string_printf : Raptor_lib/Strings/raptor_string_printf  formatString='%u'
  y_end_offset : Outport  VectorParamsAs1DForOutWhenUnconnected=off
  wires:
  raptor_string/1 -> raptor_string_printf/1
  Add22/1 -> display_draw_text13/2, y_end_offset/1, display_draw_text14/2
  In3/1 -> display_draw_text14/1
  raptor_string_printf/1 -> display_draw_text14/3
  y_start_offset/1 -> Add22/1
  Constant26/1 -> Add22/2
  in_value/1 -> raptor_string_printf/2
  x/1 -> display_draw_text13/1

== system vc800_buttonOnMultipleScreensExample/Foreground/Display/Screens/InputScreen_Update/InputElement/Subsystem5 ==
  y_start_offset : Inport
  x : Inport  Port=2
  In3 : Inport  Port=3
  in_value : Inport  Port=4
  Add22 : Sum
  Constant26 : Constant  Value=40  OutDataTypeStr=int32
  display_draw_text13 : Raptor_display_lib/Drawing Functions/display_draw_text  textPort=off  textVal=in_nam  colorPort=off  col=FFFF  opacity=100  font=Future  fontFile=''  heightPort=off  height=20  hAlign=Right  vAlign=Center  spacing=0  layer=Background  pnPort=off
  display_draw_text14 : Raptor_display_lib/Drawing Functions/display_draw_text  textPort=on  textVal='Input1'  colorPort=off  col=FFFF  opacity=100  font=Future  fontFile=''  heightPort=off  height=20  hAlign=Left  vAlign=Center  spacing=0  layer=Background  pnPort=off
  raptor_string : Raptor_lib/Strings/raptor_string  stringName=''  string=''  dynamicSize=Fixed Size  strSize=10  storage=Volatile (RAM)  calVisible=off  calAccess=4  strFunction=raptor_xcp_function(gcb)
  raptor_string_printf : Raptor_lib/Strings/raptor_string_printf  formatString='%u'
  y_end_offset : Outport  VectorParamsAs1DForOutWhenUnconnected=off
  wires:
  x/1 -> display_draw_text13/1
  in_value/1 -> raptor_string_printf/2
  Constant26/1 -> Add22/2
  y_start_offset/1 -> Add22/1
  raptor_string_printf/1 -> display_draw_text14/3
  In3/1 -> display_draw_text14/1
  Add22/1 -> display_draw_text14/2, y_end_offset/1, display_draw_text13/2
  raptor_string/1 -> raptor_string_printf/1

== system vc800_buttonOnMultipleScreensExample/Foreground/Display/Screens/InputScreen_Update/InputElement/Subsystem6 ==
  y_start_offset : Inport
  x : Inport  Port=2
  In3 : Inport  Port=3
  in_value : Inport  Port=4
  Add22 : Sum
  Constant26 : Constant  Value=40  OutDataTypeStr=int32
  display_draw_text13 : Raptor_display_lib/Drawing Functions/display_draw_text  textPort=off  textVal=in_nam  colorPort=off  col=FFFF  opacity=100  font=Future  fontFile=''  heightPort=off  height=20  hAlign=Right  vAlign=Center  spacing=0  layer=Background  pnPort=off
  display_draw_text14 : Raptor_display_lib/Drawing Functions/display_draw_text  textPort=on  textVal='Input1'  colorPort=off  col=FFFF  opacity=100  font=Future  fontFile=''  heightPort=off  height=20  hAlign=Left  vAlign=Center  spacing=0  layer=Background  pnPort=off
  raptor_string : Raptor_lib/Strings/raptor_string  stringName=''  string=''  dynamicSize=Fixed Size  strSize=10  storage=Volatile (RAM)  calVisible=off  calAccess=4  strFunction=raptor_xcp_function(gcb)
  raptor_string_printf : Raptor_lib/Strings/raptor_string_printf  formatString='%u'
  y_end_offset : Outport  VectorParamsAs1DForOutWhenUnconnected=off
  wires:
  raptor_string/1 -> raptor_string_printf/1
  Add22/1 -> display_draw_text13/2, y_end_offset/1, display_draw_text14/2
  In3/1 -> display_draw_text14/1
  raptor_string_printf/1 -> display_draw_text14/3
  y_start_offset/1 -> Add22/1
  Constant26/1 -> Add22/2
  in_value/1 -> raptor_string_printf/2
  x/1 -> display_draw_text13/1

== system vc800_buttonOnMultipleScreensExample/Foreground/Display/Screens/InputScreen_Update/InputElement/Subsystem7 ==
  y_start_offset : Inport
  x : Inport  Port=2
  In3 : Inport  Port=3
  in_value : Inport  Port=4
  Add22 : Sum
  Constant26 : Constant  Value=40  OutDataTypeStr=int32
  display_draw_text13 : Raptor_display_lib/Drawing Functions/display_draw_text  textPort=off  textVal=in_nam  colorPort=off  col=FFFF  opacity=100  font=Future  fontFile=''  heightPort=off  height=20  hAlign=Right  vAlign=Center  spacing=0  layer=Background  pnPort=off
  display_draw_text14 : Raptor_display_lib/Drawing Functions/display_draw_text  textPort=on  textVal='Input1'  colorPort=off  col=FFFF  opacity=100  font=Future  fontFile=''  heightPort=off  height=20  hAlign=Left  vAlign=Center  spacing=0  layer=Background  pnPort=off
  raptor_string : Raptor_lib/Strings/raptor_string  stringName=''  string=''  dynamicSize=Fixed Size  strSize=10  storage=Volatile (RAM)  calVisible=off  calAccess=4  strFunction=raptor_xcp_function(gcb)
  raptor_string_printf : Raptor_lib/Strings/raptor_string_printf  formatString='%u'
  y_end_offset : Outport  VectorParamsAs1DForOutWhenUnconnected=off
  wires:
  raptor_string/1 -> raptor_string_printf/1
  Add22/1 -> display_draw_text13/2, y_end_offset/1, display_draw_text14/2
  In3/1 -> display_draw_text14/1
  raptor_string_printf/1 -> display_draw_text14/3
  y_start_offset/1 -> Add22/1
  Constant26/1 -> Add22/2
  in_value/1 -> raptor_string_printf/2
  x/1 -> display_draw_text13/1

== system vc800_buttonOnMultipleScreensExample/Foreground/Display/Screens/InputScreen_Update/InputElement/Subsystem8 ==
  y_start_offset : Inport
  x : Inport  Port=2
  In3 : Inport  Port=3
  in_value : Inport  Port=4
  Add22 : Sum
  Constant26 : Constant  Value=40  OutDataTypeStr=int32
  display_draw_text13 : Raptor_display_lib/Drawing Functions/display_draw_text  textPort=off  textVal=in_nam  colorPort=off  col=FFFF  opacity=100  font=Future  fontFile=''  heightPort=off  height=20  hAlign=Right  vAlign=Center  spacing=0  layer=Background  pnPort=off
  display_draw_text14 : Raptor_display_lib/Drawing Functions/display_draw_text  textPort=on  textVal='Input1'  colorPort=off  col=FFFF  opacity=100  font=Future  fontFile=''  heightPort=off  height=20  hAlign=Left  vAlign=Center  spacing=0  layer=Background  pnPort=off
  raptor_string : Raptor_lib/Strings/raptor_string  stringName=''  string=''  dynamicSize=Fixed Size  strSize=10  storage=Volatile (RAM)  calVisible=off  calAccess=4  strFunction=raptor_xcp_function(gcb)
  raptor_string_printf : Raptor_lib/Strings/raptor_string_printf  formatString='%u'
  y_end_offset : Outport  VectorParamsAs1DForOutWhenUnconnected=off
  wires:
  x/1 -> display_draw_text13/1
  in_value/1 -> raptor_string_printf/2
  Constant26/1 -> Add22/2
  y_start_offset/1 -> Add22/1
  raptor_string_printf/1 -> display_draw_text14/3
  In3/1 -> display_draw_text14/1
  Add22/1 -> display_draw_text14/2, y_end_offset/1, display_draw_text13/2
  raptor_string/1 -> raptor_string_printf/1
